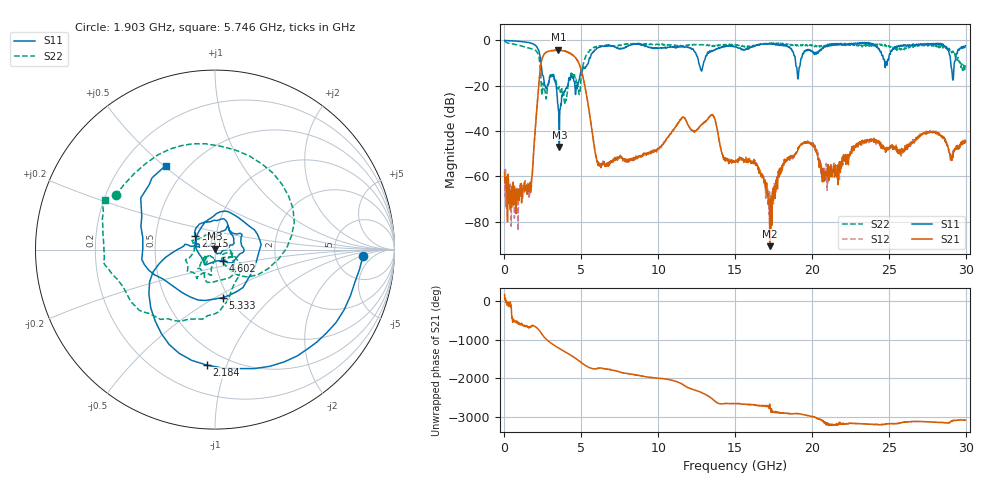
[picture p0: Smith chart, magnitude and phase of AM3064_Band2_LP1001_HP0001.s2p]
# Hz S DB R 50.0
!freq dBS11 angS11 dBS21 angS21 dBS12 angS12 dBS22 angS22
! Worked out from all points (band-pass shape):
!   1600 points, 10 MHz to 29.98 GHz, reference 50 ohm
!   highest |S21| = -4.14 dB at 3.515 GHz (marker M1); lowest = -90.9 dB at 17.25 GHz (marker M2)
!   |S21| within 3 dB of the highest: 2.498 GHz to 4.56 GHz (2.063 GHz wide, 58.5 % of centre)
!   lowest |S11| = -47.1 dB at 3.571 GHz (marker M3), VSWR 1.01, Z = 50 + j0.443 ohm
!   |S11| at or under -10 dB: 2.374 GHz to 5.451 GHz (3.077 GHz wide, 78.6 % of centre); 12.64 GHz to 12.95 GHz (310.3 MHz wide, 2.43 % of centre); 18.94 GHz to 19.25 GHz (305.1 MHz wide, 1.6 % of centre)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
!   |S22| runs from -28.2 to -0.3 dB; largest |S21 - S12| = 0.015
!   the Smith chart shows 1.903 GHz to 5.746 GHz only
!   S11 on the Smith chart (normalised r, x): 1.903 GHz: 10, -2; 2.184 GHz: 0.39, -0.85; 2.915 GHz: 0.79, +0.12; 4.602 GHz: 1.08, -0.13; 5.333 GHz: 0.94, -0.54; 5.746 GHz: 0.38, +0.51
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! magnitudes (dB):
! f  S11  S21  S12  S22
! 10 MHz  0.0  -58.4  -56.8  -0.3
! 1.603 GHz  -1.0  -66.8  -69.8  -3.4
! 1.903 GHz  -1.7  -48.5  -48.5  -4.0
! 2.184 GHz  -3.8  -23.6  -23.5  -5.9
! 2.559 GHz  -17.1  -6.3  -6.3  -20.5
! 2.915 GHz  -17.4  -4.7  -4.7  -16.7
! 3.515 GHz  -31.0  -4.1  -4.2  -21.5
! 3.571 GHz  -47.1  -4.2  -4.2  -20.4
! 4.602 GHz  -22.4  -7.5  -7.4  -17.6
! 5.015 GHz  -13.0  -13.5  -13.6  -14.9
! 5.333 GHz  -11.3  -23.8  -23.9  -6.1
! 5.746 GHz  -5.3  -42.3  -42.3  -3.4
! 6.252 GHz  -2.8  -55.0  -55.3  -2.4
! 10 GHz  -3.4  -47.9  -47.5  -1.8
! 13.49 GHz  -4.5  -33.1  -32.9  -2.3
! 15 GHz  -2.6  -53.5  -53.6  -1.8
! 16.39 GHz  -2.1  -55.0  -53.7  -2.3
! 17.25 GHz  -1.4  -90.9  -67.1  -1.2
! 19.99 GHz  -4.6  -46.0  -46.3  -1.9
! 20.8 GHz  -2.7  -62.2  -56.0  -2.6
! 25 GHz  -8.0  -47.8  -48.4  -2.3
! 29.98 GHz  -2.4  -44.4  -45.4  -10.9
